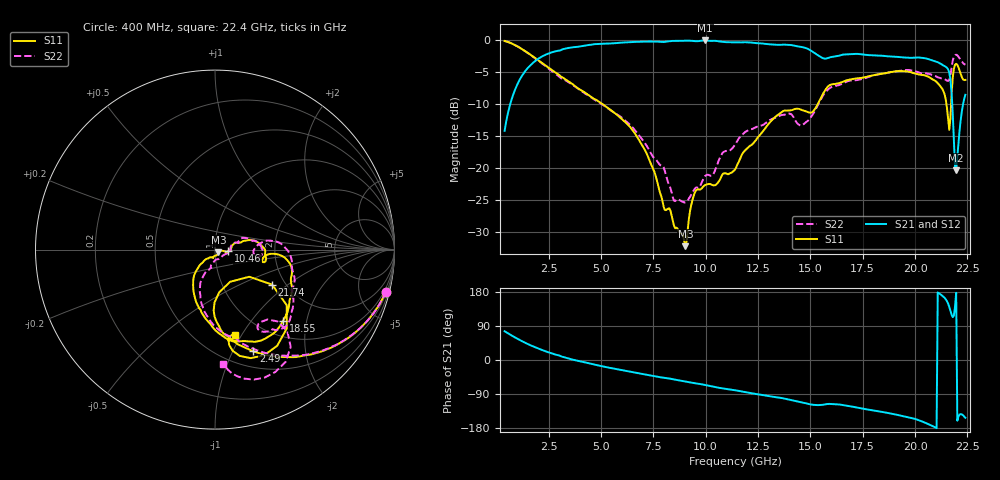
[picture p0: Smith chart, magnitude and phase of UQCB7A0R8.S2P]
!  Part Number  UQCB7A0R8	Mounting Orientation: Vertical
!  Description: RF capacitors
!  Application: Coupling, Bypass, Tuning, DC Block
!  Filters, Matching
# GHZ S DB R 50
! Freq  |S11|  S11 Ph  |S21|  S21 Ph  |S12|  S12 Ph  |S22|  S22 Ph
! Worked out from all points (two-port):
!   401 points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, 400 MHz to 22.4 GHz, reference 50 ohm
!   highest |S21| = -0.10 dB at 9.97 GHz (marker M1); lowest = -20.4 dB at 21.96 GHz (marker M2)
!   |S21| within 3 dB of the highest: 1.944 GHz to 20.72 GHz (18.77 GHz wide, 166 % of centre)
!   lowest |S11| = -32.2 dB at 9.035 GHz (marker M3), VSWR 1.05, Z = 51.9 - j1.62 ohm
!   |S11| at or under -10 dB: 5.055 GHz to 15.36 GHz (10.3 GHz wide, 101 % of centre); 21.49 GHz to 21.72 GHz (226.2 MHz wide, 1.05 % of centre)
!   |S22| runs from -25.4 to -0.2 dB; largest |S21 - S12| = 0.0043
!   S11 on the Smith chart (normalised r, x): 400 MHz: 0.69, -8.09; 2.49 GHz: 0.67, -1.21; 10.46 GHz: 1.16, -0.02; 18.55 GHz: 1.29, -1.46; 21.74 GHz: 1.71, -0.78; 22.4 GHz: 0.75, -0.93
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0.4  -0.18 -14.0  -14.22 75.9  -14.23 75.9  -0.17 -13.8
1.17  -1.32 -38.4  -5.94 51.4  -5.95 51.4  -1.32 -38.1
2.49  -4.35 -69.3  -2.15 20.4  -2.15 20.3  -4.48 -68.4
4.085  -7.93 -95.6  -0.99 -4.4  -0.99 -4.4  -8.05 -94.0
6.45  -13.86 -126.5  -0.35 -31.3  -0.35 -31.3  -13.47 -112.9
7.77  -23.29 -131.9  -0.29 -44.9  -0.29 -44.9  -19.36 -104.2
8.485  -29.01 -93.6  -0.17 -51.3  -0.17 -51.3  -25.11 -82.6
9.035  -32.24 -39.6  -0.14 -56.9  -0.14 -56.9  -25.39 -42.9
9.42  -24.45 -11.7  -0.18 -60.9  -0.18 -60.9  -23.57 -20.2
9.97  -22.70 -15.6  -0.10 -66.1  -0.10 -66.1  -21.30 -2.2
10.465  -22.72 -7.4  -0.16 -71.5  -0.16 -71.5  -20.26 15.8
11.4  -20.27 12.6  -0.38 -79.8  -0.38 -79.8  -16.40 22.4
13.49  -11.63 4.5  -0.79 -99.2  -0.79 -99.2  -11.95 5.8
15.085  -11.31 -9.6  -1.81 -118.0  -1.81 -117.9  -11.81 8.1
15.965  -7.02 -15.9  -2.71 -116.0  -2.75 -116.1  -7.46 -5.2
18.55  -5.23 -46.2  -2.53 -138.3  -2.51 -138.3  -5.23 -38.4
18.77  -5.08 -49.0  -2.59 -140.6  -2.58 -140.7  -5.08 -39.7
21.08  -6.77 -85.1  -3.50 178.2  -3.49 178.1  -5.85 -61.4
21.52  -10.62 -90.5  -4.36 155.1  -4.36 155.1  -6.38 -59.6
21.74  -8.56 -31.5  -8.21 119.7  -8.20 119.5  -4.33 -48.5
21.96  -3.75 -65.1  -20.36 177.3  -20.40 176.8  -2.33 -69.0
22.4  -6.26 -76.8  -8.59 -152.5  -8.53 -152.7  -3.88 -85.8
